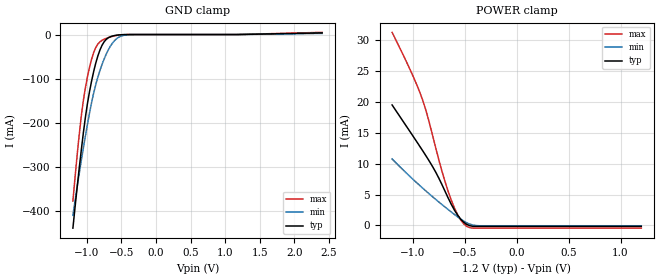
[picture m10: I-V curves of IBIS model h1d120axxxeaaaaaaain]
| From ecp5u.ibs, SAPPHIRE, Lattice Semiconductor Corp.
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|   Model h1d120axxxeaaaaaaain
[Model] h1d120axxxeaaaaaaain
Model_type Input
Polarity   Non-Inverting
Vinl =  0.500V
Vinh =  0.700V
C_comp   3.899pF   3.899pF   3.904pF
[Temperature Range]   25.000   0.125k   -40.000
[Voltage Range]   1.200V   1.140V   1.260V
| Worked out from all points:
|   GND clamp passes 1 mA (typ) near -0.54 V on its own axis
|   POWER clamp passes 1 mA (typ) near -0.54 V on its own axis
[GND_clamp]
|Voltage   I(typ)   I(min)   I(max)
-1.2V     -438mA     -409.1mA   -376.6mA
-1.14V    -347.3mA   -346mA     -275mA
-1.08V    -262.9mA   -286.2mA   -186mA
-1.05V    -223.7mA   -257.7mA   -150.1mA
-990mV    -156.2mA   -203.2mA   -95.71mA
-900mV    -83.64mA   -132.1mA   -40.81mA
-840mV    -48.61mA   -96.59mA   -21.71mA
-780mV    -24.63mA   -67.99mA   -13.11mA
-690mV    -7.398mA   -35.03mA   -7.025mA
-570mV    -1.527mA   -9.488mA   -1.957mA
-420mV    -83.23uA   -670.2uA   -76.79uA
2.4V      3.704mA    2.56mA     4.906mA
[POWER_clamp]
|Voltage   I(typ)   I(min)   I(max)
-1.2V     19.53mA    10.77mA    31.3mA
-990mV    14.26mA    7.336mA    23.89mA
-900mV    11.96mA    5.959mA    20.04mA
-840mV    10.37mA    5.073mA    16.56mA
-720mV    6.62mA     3.379mA    8.8mA
-660mV    4.443mA    2.57mA     5.508mA
-630mV    3.417mA    2.174mA    4.085mA
-570mV    1.681mA    1.398mA    1.76mA
-540mV    1.015mA    1.031mA    892.9uA
-480mV    148.6uA    407.1uA    -173.6uA
-360mV    -173.8uA   -61.24uA   -447.3uA
1.2V      -173.8uA   -65.23uA   -447.3uA
